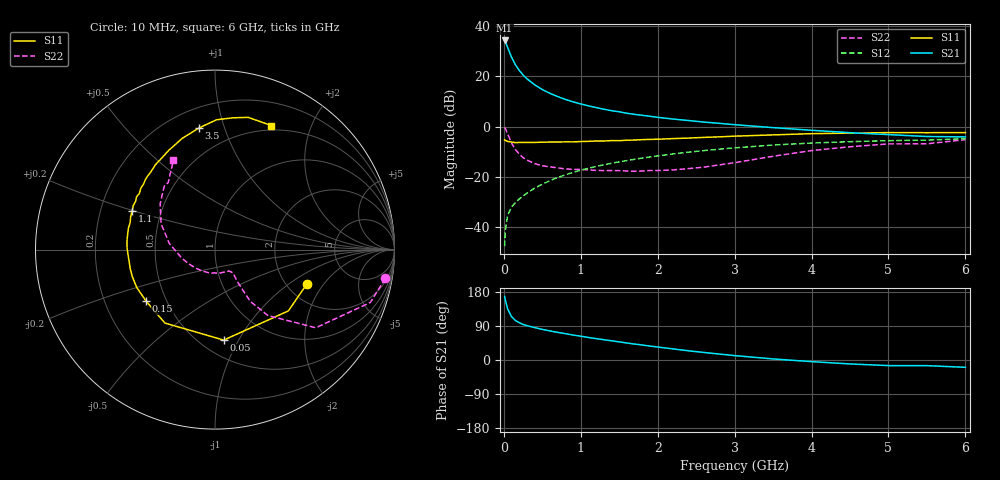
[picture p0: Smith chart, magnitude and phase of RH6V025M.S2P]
! SIEMENS Small Signal Semiconductors
! BFR106
! Si NPN RF Bipolar Junction Transistor in SOT23
! VCE = 6 V  IC = 25 mA
! Common Emitter S-Parameters:  August  1996
# GHz  S  MA  R  50
!  f  S11  S21  S12  S22
! GHz  MAG  ANG  MAG  ANG  MAG  ANG  MAG  ANG
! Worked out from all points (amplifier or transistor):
!   36 points, 10 MHz to 6 GHz, reference 50 ohm
!   highest |S21| = 34.2 dB at 10 MHz (marker M1)
!   |S21| within 3 dB of that: start of sweep to 51.8 MHz
!   unconditionally stable (mu >= 1): 345.4 MHz to 2.13 GHz
!   at 250 MHz: K = 0.92, MSG = 24.1 dB, |S12| = -27.6 dB
!   at 1.4 GHz: K = 1.06, MAG = 8.9 dB, |S12| = -14.6 dB
!   at 6 GHz: K = 0.99, MSG = 0.4 dB, |S12| = -4.8 dB
!   S11 on the Smith chart (normalised r, x): 10 MHz: 2.54, -1.39; 50 MHz: 0.64, -0.87; 150 MHz: 0.39, -0.29; 1.1 GHz: 0.34, +0.20; 3.5 GHz: 0.32, +0.83; 6 GHz: 0.45, +1.46
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0.01  0.5463 -20.6  51.53 167.6  0.0042 82.9  0.9623 -9.6
0.02  0.5327 -39.9  48.7 157.6  0.0088 75.5  0.9142 -18.8
0.05  0.5064 -84.5  37.06 134.2  0.0173 61.4  0.7107 -37.8
0.1  0.4954 -124.3  23.98 114.6  0.0253 55.5  0.4715 -51.2
0.15  0.4793 -143.0  16.99 104.2  0.0307 56.4  0.35 -55.7
0.2  0.4843 -154.0  13.13 98.5  0.0364 59.4  0.2854 -55.5
0.25  0.4846 -161.7  10.61 93.8  0.0416 61.3  0.2413 -55.3
0.3  0.4841 -166.9  8.925 90.7  0.0474 63.5  0.2169 -55.1
0.4  0.4846 -175.7  6.782 85.5  0.0598 66.2  0.1841 -53.5
0.5  0.4897 179.3  5.445 80.8  0.0716 67.6  0.1666 -52.5
0.6  0.493 174.1  4.569 76.7  0.0847 67.9  0.1584 -53.1
0.7  0.494 170.0  3.952 72.8  0.0973 68.1  0.1511 -54.8
0.9  0.496 162.4  3.104 65.9  0.1231 67.1  0.1411 -57.8
1.1  0.5092 154.8  2.583 59.4  0.1486 65.8  0.1379 -65.1
1.3  0.5177 148.8  2.216 53.5  0.1741 63.8  0.1336 -71.9
1.6  0.536 140.5  1.844 44.8  0.2115 60.4  0.1311 -85.9
2.2  0.5776 125.1  1.411 29.3  0.2864 52.8  0.1377 -119.1
2.8  0.625 110.8  1.161 15.7  0.3557 44.2  0.1734 -156.4
3.5  0.6839 97.4  0.954 2.8  0.4297 33.8  0.2574 172.1
4.5  0.7412 82.2  0.757 -10.4  0.501 18.4  0.3972 140.3
5.5  0.7564 69.9  0.635 -14.9  0.5386 7.9  0.455 125.0
6  0.7589 65.6  0.624 -19.3  0.575 0.4  0.5501 114.9
